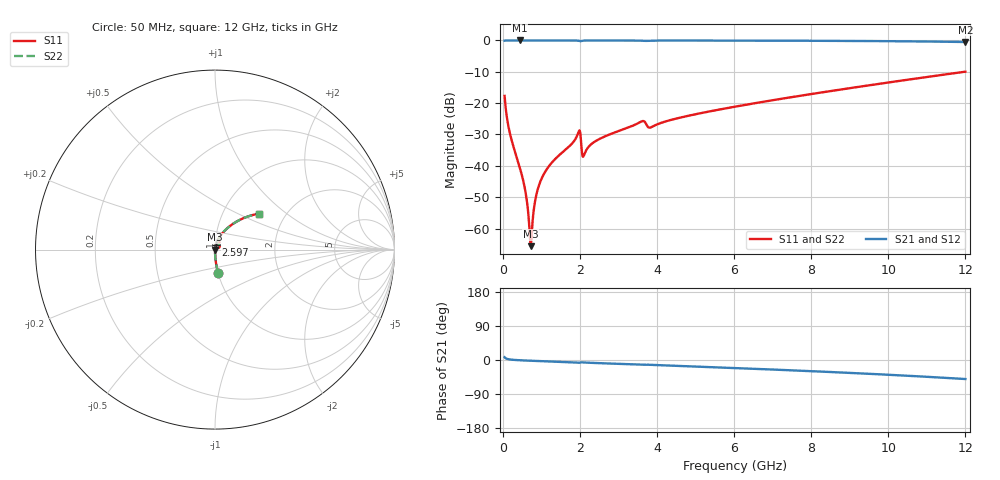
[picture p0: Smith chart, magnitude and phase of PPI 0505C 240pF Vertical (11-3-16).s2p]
# GHz S MA R 50
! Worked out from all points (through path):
!   1601 points, 50 MHz to 12 GHz, reference 50 ohm
!   highest |S21| = 0.00 dB at 445.8 MHz (marker M1); lowest = -0.5 dB at 12 GHz (marker M2)
!   group delay of S21, straight-line fit = 11.5 ps
!   lowest |S11| = -65.6 dB at 729.7 MHz (marker M3), VSWR 1.00, Z = 50.1 + j0.00492 ohm
!   |S11| at or under -10 dB: start of sweep to 11.98 GHz
!   |S22| runs from -65.6 to -10.0 dB; largest |S21 - S12| = 0
!   S11 on the Smith chart (normalised r, x): 50 MHz: 1.00, -0.26; 2.597 GHz: 1.01, +0.06; 12 GHz: 1.48, +0.66
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0.05  0.1307 -82.5  0.9912 7.4  0.9912 7.4  0.1307 -82.5
0.1919063  0.03211 -88.1  0.9992 1.3  0.9992 1.3  0.03211 -88.1
0.4458437  0.009313 -88.0  0.9995 -0.7  0.9995 -0.7  0.009313 -88.0
0.5802812  0.004197 -84.8  0.9995 -1.3  0.9995 -1.3  0.004197 -84.8
0.6848437  0.001211 -67.1  0.9994 -1.8  0.9994 -1.8  0.001211 -67.1
0.7296563  0.0005236 5.4  0.9994 -2.0  0.9994 -2.0  0.0005236 5.4
0.767  0.001121 59.7  0.9994 -2.1  0.9994 -2.1  0.001121 59.7
0.8342188  0.00261 75.5  0.9994 -2.4  0.9994 -2.4  0.00261 75.5
0.8939687  0.003902 79.0  0.9994 -2.6  0.9994 -2.6  0.003902 79.0
1.103094  0.008073 82.1  0.9993 -3.5  0.9993 -3.5  0.008073 82.1
1.954531  0.03312 68.3  0.991 -7.1  0.991 -7.1  0.03312 68.3
2.044156  0.01955 26.0  0.9833 -6.1  0.9833 -6.1  0.01955 26.0
2.118844  0.01534 67.0  0.9954 -6.6  0.9954 -6.6  0.01534 67.0
2.290625  0.022 78.6  0.9981 -7.5  0.9981 -7.5  0.022 78.6
2.596844  0.02848 79.1  0.9983 -8.7  0.9983 -8.7  0.02848 79.1
3.605125  0.05122 69.1  0.9911 -12.7  0.9911 -12.7  0.05122 69.1
3.81425  0.04069 65.8  0.9908 -12.6  0.9908 -12.6  0.04069 65.8
4.038312  0.04671 73.3  0.9961 -13.6  0.9961 -13.6  0.04671 73.3
6.025  0.08786 67.8  0.9942 -21.3  0.9942 -21.3  0.08786 67.8
8.019156  0.1402 59.7  0.9877 -29.5  0.9877 -29.5  0.1402 59.7
10.01331  0.214 50.4  0.9738 -39.0  0.9738 -39.0  0.214 50.4
12  0.3177 39.2  0.9441 -50.2  0.9441 -50.2  0.3177 39.2
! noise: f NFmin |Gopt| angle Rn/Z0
0.05  0.000325  0.8398  0.2513  0.0004299
1.372  0.003189  0.6085  3.631  0.001507
2.701  0.005618  0.5727  7.044  0.002372
4.031  0.01043  0.6423  10.63  0.005469
5.36  0.009189  0.5063  13.43  0.003188
6.682  0.01091  0.4894  16.36  0.003597
8.012  0.01292  0.4868  19.24  0.004203
9.341  0.01522  0.4932  22.04  0.004996
10.67  0.01791  0.5073  24.81  0.006046
12  0.02114  0.5286  27.58  0.007485
